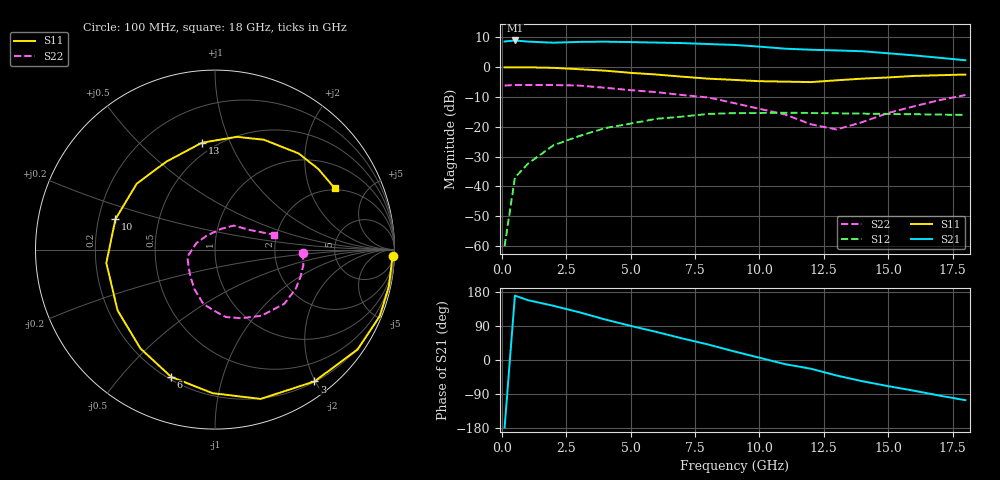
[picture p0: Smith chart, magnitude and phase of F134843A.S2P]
!ATF-13484
!S-PARAMETERS at Vds=2.5V  Id=20mA.  LAST UPDATED 07-22-92
# ghz s ma r 50
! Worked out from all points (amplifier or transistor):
!   20 points, 100 MHz to 18 GHz, reference 50 ohm
!   highest |S21| = 8.9 dB at 500 MHz (marker M1)
!   |S21| within 3 dB of that: start of sweep to 11.68 GHz
!   unconditionally stable (mu >= 1): start of sweep to 260.1 MHz; 10.51 GHz to end of sweep
!   at 2 GHz: K = 0.26, MSG = 17.2 dB, |S12| = -26.2 dB
!   at 9 GHz: K = 0.87, MSG = 11.4 dB, |S12| = -15.4 dB
!   at 18 GHz: K = 1.19, MAG = 6.5 dB, |S12| = -16.0 dB
!   lowest NFmin = 0.80 dB at 500 MHz
!   S11 on the Smith chart (normalised r, x): 100 MHz: 15, -53; 3 GHz: 0.21, -1.99; 6 GHz: 0.21, -0.69; 10 GHz: 0.27, +0.14; 13 GHz: 0.42, +0.79; 18 GHz: 1.94, +3.01
0.1  0.99 -2.0  2.68 -178.0  0.001 95.0  0.49 -2.0
0.5  0.99 -12.0  2.79 170.0  0.014 81.0  0.5 -10.0
1  0.99 -22.0  2.67 158.0  0.024 78.0  0.5 -18.0
2  0.97 -35.0  2.56 143.0  0.049 63.0  0.5 -26.0
3  0.92 -53.0  2.64 126.0  0.07 51.0  0.49 -38.0
4  0.87 -73.0  2.66 107.0  0.095 38.0  0.45 -55.0
5  0.8 -91.0  2.62 90.0  0.113 28.0  0.41 -69.0
6  0.75 -109.0  2.57 74.0  0.136 16.0  0.38 -81.0
7  0.69 -127.0  2.52 57.0  0.148 5.0  0.34 -91.0
8  0.64 -148.0  2.43 41.0  0.164 -5.0  0.31 -102.0
9  0.61 -173.0  2.35 23.0  0.169 -14.0  0.25 -117.0
10  0.58 163.0  2.2 6.0  0.17 -28.0  0.2 -134.0
11  0.57 140.0  2.03 -11.0  0.172 -38.0  0.16 -165.0
12  0.56 119.0  1.95 -23.0  0.17 -49.0  0.11 161.0
13  0.6 97.0  1.9 -41.0  0.168 -59.0  0.09 121.0
14  0.64 79.0  1.84 -56.0  0.166 -75.0  0.12 74.0
15  0.67 66.0  1.7 -69.0  0.164 -79.0  0.17 52.0
16  0.71 49.0  1.57 -81.0  0.162 -82.0  0.22 30.0
17  0.73 38.0  1.43 -94.0  0.16 -85.0  0.28 20.0
18  0.75 27.0  1.3 -106.0  0.158 -89.0  0.34 14.0
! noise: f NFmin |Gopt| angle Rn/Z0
0.5  0.8  0.96  7  1.3
1  0.8  0.92  14  1.3
2  0.8  0.85  28  1.1
4  1  0.76  61  0.9
6  1.2  0.68  105  0.6
8  1.5  0.6  152  0.2
12  2  0.55  -104  0.2
15  2.8  0.6  -37  0.6
